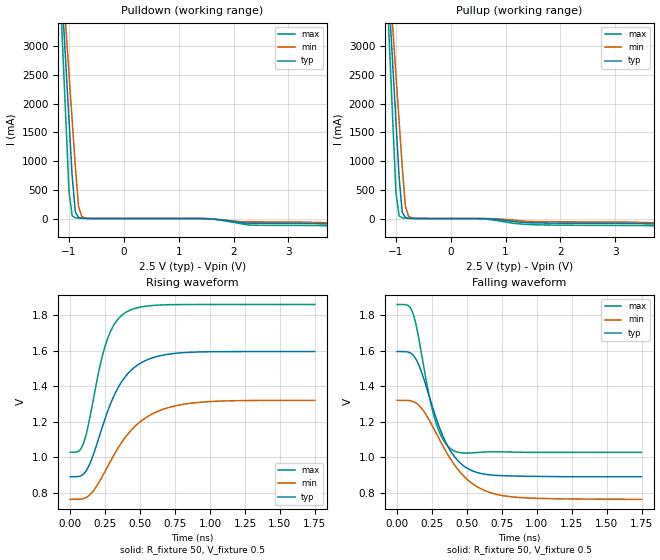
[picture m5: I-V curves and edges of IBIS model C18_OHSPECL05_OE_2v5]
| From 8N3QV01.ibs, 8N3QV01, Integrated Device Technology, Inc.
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[Model] C18_OHSPECL05_OE_2v5
Model_type   Output_ECL
Polarity   Non-Inverting
|   typ   min   max
C_comp   2pF   1.5pF   2.5pF
Vmeas = 1.25V
Rref = 50
Cref = 0
Vref = 0.5V
|   typ   min   max
[Voltage range]   2.5V   2.375V   2.625V
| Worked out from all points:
|   rising waveform, R_fixture 50, V_fixture 0.5: 20-80 % time 222ps typ, 298ps min, 147ps max; typ from 0.89 V to 1.59 V
|   falling waveform, R_fixture 50, V_fixture 0.5: 20-80 % time 200ps typ, 272ps min, 129ps max; typ from 1.59 V to 0.89 V
[Pulldown]
|Voltage   I (typ)   I (min)   I (max)
-2.5V     31.14A     27.8A      36.91A
-1.3V     6.78A      6.74A      6.961A
-1V       1.716A     2.526A     483.4mA
-941.5mV  730.2mA    1.706A     45.91mA
-884.1mV  108.8mA    899.7mA    12.51mA
-826.6mV  20.14mA    210.5mA    6.917mA
-769.2mV  5.982mA    41.46mA    4.556mA
-711.7mV  2.46mA     10.05mA    2.781mA
1.472V    -1.209mA   -1.638mA   -1.061mA
2.276V    -80.57mA   -56.82mA   -112.8mA
3.655V    -92.97mA   -70.89mA   -125.2mA
5V        -139.4mA   -107.3mA   -188.7mA
[Pullup]
|Voltage   I (typ)   I (min)   I (max)
-2.5V     31.14A     27.8A      36.91A
-1.3V     6.78A      6.74A      6.961A
-1V       1.716A     2.526A     483.4mA
-941.5mV  730.2mA    1.706A     45.91mA
-884.1mV  108.8mA    899.7mA    12.51mA
-826.6mV  20.14mA    210.5mA    6.917mA
-769.2mV  5.982mA    41.46mA    4.556mA
-711.7mV  2.46mA     10.05mA    2.781mA
495mV     -87.68uA   -7.314uA   -990.8uA
1.472V    -73.59mA   -51.46mA   -105.4mA
3.598V    -91.45mA   -69.62mA   -123.8mA
5V        -139.3mA   -107.3mA   -188.3mA
[Ramp]
|   typ   min   max
dV/dt_r   0.562/0.353n   0.444/0.472n   0.664/0.232n
dV/dt_f   0.563/0.309n   0.445/0.422n   0.668/0.196n
R_load =   50.0000
[Rising Waveform]
R_fixture = 50
V_fixture = 0.5   | VCC_typ - 2V
V_fixture_max = 0.625   | VCC_max - 2V
V_fixture_min = 0.375   | VCC_min - 2V
C_fixture = 0.0p
| Time   typ   min   max
0s        890.5mV    763.6mV    1.028V
92.84ps   904.4mV    767.5mV    1.074V
150.7ps   983.5mV    797.8mV    1.266V
208.5ps   1.119V     863.1mV    1.499V
255.8ps   1.232V     931mV      1.641V
318.8ps   1.356V     1.022V     1.752V
397.6ps   1.457V     1.116V     1.815V
562.3ps   1.552V     1.233V     1.851V
783ps     1.586V     1.294V     1.858V
1.748ns   1.594V     1.32V      1.859V
[Falling Waveform]
R_fixture = 50
V_fixture = 0.5   | VCC_typ - 2V
V_fixture_max = 0.625   | VCC_max - 2V
V_fixture_min = 0.375   | VCC_min - 2V
C_fixture = 0.0p
| Time   typ   min   max
0s        1.594V     1.32V      1.859V
110.4ps   1.577V     1.314V     1.815V
168.2ps   1.493V     1.281V     1.61V
224.2ps   1.356V     1.217V     1.365V
268ps     1.246V     1.153V     1.22V
325.8ps   1.122V     1.066V     1.103V
395.9ps   1.019V     973.1mV    1.041V
529ps     926.9mV    857.2mV    1.025V
735.7ps   896.9mV    787.5mV    1.031V
1.748ns   890.5mV    763.6mV    1.028V
